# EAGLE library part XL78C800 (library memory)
MEMORY
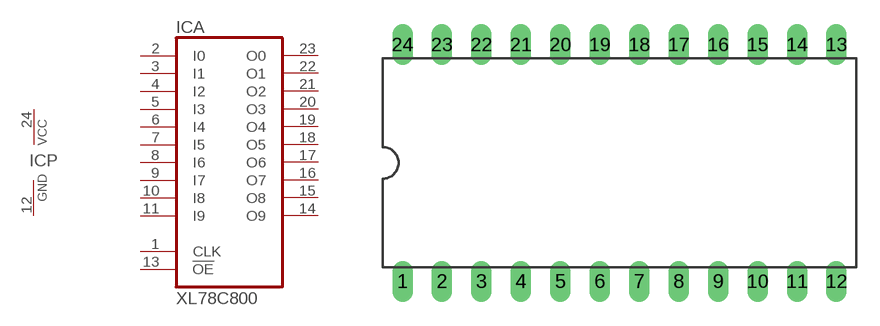
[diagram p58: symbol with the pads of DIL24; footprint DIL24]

Designator prefix IC; gates A=XL78C800 P=PWRN

## XL78C800  [DIL24]
1  A:CLK  in
2  A:I0  in
3  A:I1  in
4  A:I2  in
5  A:I3  in
6  A:I4  in
7  A:I5  in
8  A:I6  in
9  A:I7  in
10  A:I8  in
11  A:I9  in
12  P:GND  pwr
13  A:!OE  in
14  A:O9
15  A:O8  hiz
16  A:O7  hiz
17  A:O6  hiz
18  A:O5  hiz
19  A:O4  hiz
20  A:O3  hiz
21  A:O2  hiz
22  A:O1  hiz
23  A:O0
24  P:VCC  pwr

## Footprint DIL24 (pad centres in mm)
Dual In Line Package
drill 0.813 long: 1 -13.97,-7.62; 2 -11.43,-7.62; 3 -8.89,-7.62; 4 -6.35,-7.62; 5 -3.81,-7.62; 6 -1.27,-7.62; 7 1.27,-7.62; 8 3.81,-7.62; 9 6.35,-7.62; 10 8.89,-7.62; 11 11.43,-7.62; 12 13.97,-7.62; 13 13.97,7.62; 14 11.43,7.62; 15 8.89,7.62; 16 6.35,7.62; 17 3.81,7.62; 18 1.27,7.62; 19 -1.27,7.62; 20 -3.81,7.62; 21 -6.35,7.62; 22 -8.89,7.62; 23 -11.43,7.62; 24 -13.97,7.62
